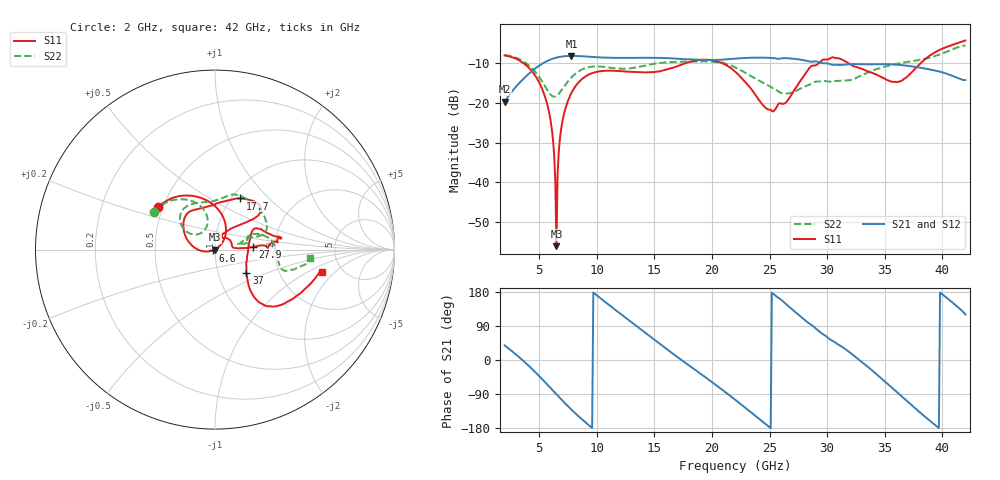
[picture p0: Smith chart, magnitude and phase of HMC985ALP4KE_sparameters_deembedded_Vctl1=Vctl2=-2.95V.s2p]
!s2p File: Measurements: S11, S21, S12, S22
# GHz S dB R 50.0
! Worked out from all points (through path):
!   401 points, 2 GHz to 42 GHz, reference 50 ohm
!   highest |S21| = -8.16 dB at 7.8 GHz (marker M1); lowest = -19.7 dB at 2 GHz (marker M2)
!   lowest |S11| = -56.1 dB at 6.5 GHz (marker M3), VSWR 1.00, Z = 49.8 + j0.0265 ohm
!   |S11| at or under -10 dB: 3.638 GHz to 17.69 GHz (14.05 GHz wide, 132 % of centre); 20.9 GHz to 29.27 GHz (8.374 GHz wide, 33.4 % of centre); 31.85 GHz to 38.11 GHz (6.269 GHz wide, 17.9 % of centre)
!   |S22| runs from -18.4 to -5.5 dB; largest |S21 - S12| = 0.00043
!   S11 on the Smith chart (normalised r, x): 2 GHz: 0.47, +0.26; 6.6 GHz: 0.98, -0.01; 17.7 GHz: 1.09, +0.69; 27.9 GHz: 1.53, +0.05; 37 GHz: 1.37, -0.37; 42 GHz: 3.55, -1.41
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2  -8.05 143.3  -19.71 38.6  -19.72 38.5  -7.94 148.7
5.2  -16.06 68.7  -10.23 -48.7  -10.24 -48.7  -14.34 103.5
6  -24.63 44.1  -9.06 -74.5  -9.06 -74.5  -17.94 114.8
6.2  -29.31 38.7  -8.85 -81.0  -8.85 -81.0  -18.37 121.8
6.3  -33.09 36.3  -8.76 -84.3  -8.76 -84.3  -18.42 125.8
6.5  -56.09 170.2  -8.59 -90.7  -8.59 -90.8  -18.24 133.3
6.6  -37.87 -159.6  -8.52 -94.0  -8.52 -94.0  -18.01 136.5
7  -24.95 -169.1  -8.31 -106.7  -8.31 -106.7  -16.55 145.3
7.8  -17.50 169.0  -8.16 -130.9  -8.16 -130.9  -13.58 146.4
8.7  -14.05 150.2  -8.25 -156.1  -8.25 -156.1  -11.61 138.1
12.4  -12.04 117.4  -8.66 114.0  -8.67 114.0  -11.40 96.4
15.4  -12.09 92.2  -8.67 44.3  -8.67 44.3  -9.96 73.8
17.7  -9.99 64.1  -8.99 -7.4  -8.99 -7.4  -9.60 62.3
22  -12.09 40.0  -8.85 -104.5  -8.85 -104.5  -11.03 17.6
25.2  -22.03 59.3  -8.69 177.7  -8.69 177.7  -16.13 16.4
27.9  -13.49 4.1  -9.20 109.4  -9.20 109.4  -16.05 12.0
28.7  -10.63 2.0  -9.61 91.2  -9.62 91.2  -15.02 11.7
32.4  -10.86 21.8  -10.22 9.5  -10.22 9.5  -13.89 22.4
35.4  -14.44 7.1  -10.25 -67.2  -10.26 -67.2  -10.61 14.1
37  -13.25 -36.5  -10.67 -110.2  -10.67 -110.2  -9.65 5.3
39.5  -7.06 -45.5  -11.92 -174.6  -11.92 -174.6  -8.04 -16.5
42  -4.27 -11.8  -14.23 119.8  -14.24 119.8  -5.51 -5.3
